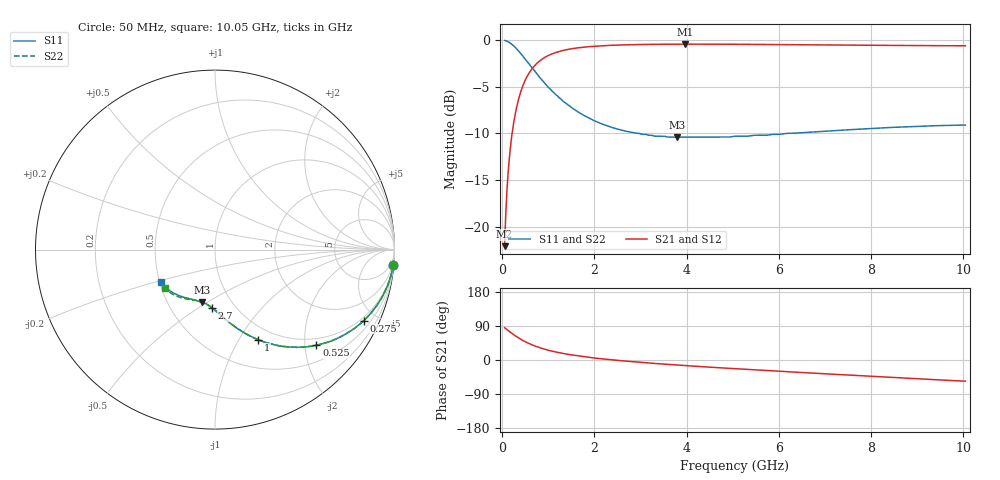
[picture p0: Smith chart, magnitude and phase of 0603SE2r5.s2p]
! AVX Thin Film Operation		Date: August 2001
! Description: Accu-P® Series, Thin Film, SMD, RF Capacitor
! Part Number: 06035J2R5ABT
! 50 MHz  -  10.05 GHz
! Serial Measurements
# mhz S db R 50
!	S11		S21		S12		S22
!	dB	Phase	dB	Phase	dB	Phase	dB	Phase
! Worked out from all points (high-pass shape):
!   401 points, 50 MHz to 10.05 GHz, reference 50 ohm
!   highest |S21| = -0.42 dB at 3.975 GHz (marker M1); lowest = -22.1 dB at 50 MHz (marker M2)
!   |S21| within 3 dB of the highest: 594.8 MHz to end of sweep
!   lowest |S11| = -10.4 dB at 3.8 GHz (marker M3), VSWR 1.87, Z = 36.7 - j23.7 ohm
!   |S11| at or under -10 dB: 2.964 GHz to 6.172 GHz (3.208 GHz wide, 70.2 % of centre)
!   |S22| runs from -10.4 to 0.0 dB; largest |S21 - S12| = 0
!   S11 on the Smith chart (normalised r, x): 50 MHz: 1, -23; 275 MHz: 0.84, -4.26; 525 MHz: 0.84, -2.25; 1 GHz: 0.83, -1.22; 2.7 GHz: 0.78, -0.57; 10.05 GHz: 0.51, -0.21
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50  -0.03 -4.9  -22.10 85.1  -22.10 85.1  -0.03 -4.9
75  -0.06 -7.3  -18.66 82.7  -18.66 82.7  -0.06 -7.3
125  -0.17 -12.1  -14.32 77.8  -14.32 77.8  -0.17 -12.1
150  -0.23 -14.5  -12.82 75.5  -12.82 75.5  -0.23 -14.5
200  -0.41 -19.1  -10.44 70.9  -10.44 70.9  -0.41 -19.1
275  -0.74 -25.5  -8.07 64.5  -8.07 64.5  -0.74 -25.5
375  -1.28 -33.3  -5.95 56.7  -5.95 56.7  -1.28 -33.3
525  -2.20 -43.4  -4.02 46.6  -4.02 46.6  -2.20 -43.4
625  -2.83 -48.9  -3.20 41.1  -3.20 41.1  -2.83 -48.9
750  -3.61 -54.9  -2.48 35.1  -2.48 35.1  -3.61 -54.8
1000  -5.06 -64.3  -1.63 25.7  -1.63 25.7  -5.06 -64.2
1350  -6.66 -73.4  -1.06 16.6  -1.06 16.6  -6.66 -73.3
1725  -7.93 -80.4  -0.77 9.6  -0.77 9.6  -7.93 -80.3
2150  -8.96 -86.8  -0.60 3.3  -0.60 3.3  -8.96 -86.5
2700  -9.78 -93.2  -0.49 -3.1  -0.49 -3.1  -9.77 -92.7
3400  -10.30 -100.3  -0.44 -9.9  -0.44 -9.9  -10.30 -99.2
3800  -10.40 -104.0  -0.42 -13.3  -0.42 -13.3  -10.40 -102.0
3975  -10.40 -105.0  -0.42 -14.7  -0.42 -14.7  -10.40 -104.0
5050  -10.30 -114.0  -0.43 -22.9  -0.43 -22.9  -10.30 -112.0
6725  -9.86 -126.0  -0.49 -34.5  -0.49 -34.5  -9.83 -123.0
8400  -9.37 -137.2  -0.56 -45.5  -0.56 -45.5  -9.34 -133.1
10050  -9.10 -148.6  -0.60 -55.9  -0.60 -55.9  -9.06 -142.8
